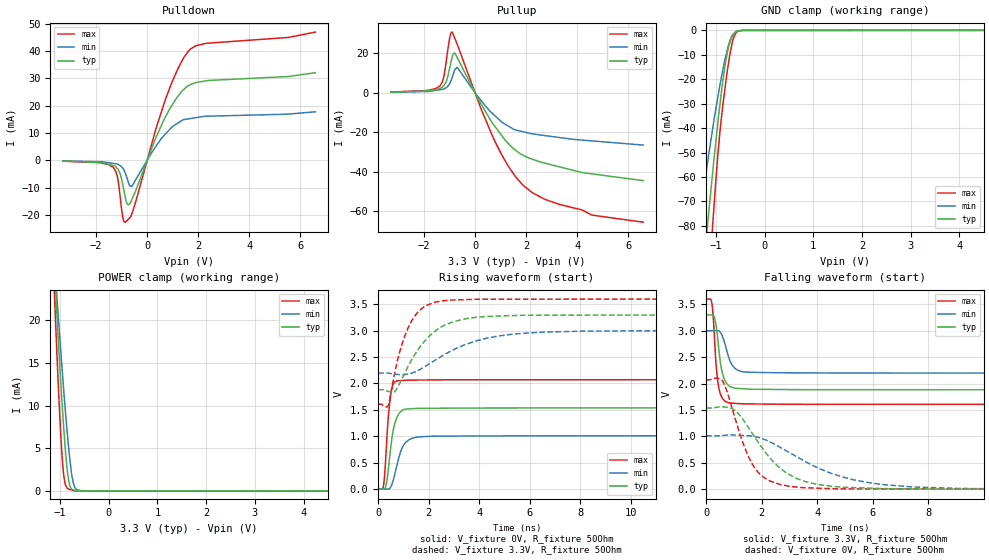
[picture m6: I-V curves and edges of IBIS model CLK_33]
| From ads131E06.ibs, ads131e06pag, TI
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|   CLK 3.3V Model
[Model]   CLK_33
Model_type   I/O
|for all products
|Signals   CLK
Vinl = 0.66
Vinh = 2.64
Vmeas = 1.65
Vref = 1.65
Cref = 2pF
Rref = 50
|   typ   min   max
|   (nom PVT)   (Fast PVT)   (slow PVT)
|C_comp from frequency sweep method (F=64MHz)
|   (HIGH Z)
|C_comp   3.0737920e-12   2.2794920e-12   3.8127910e-12
|   (ON state)
|C_comp   5.2867200e-12   4.2791250e-12   6.0292710e-12
|   (OFF state)
|C_comp   6.2204500e-12   5.1534470e-12   7.4413370e-12
|C_comp from LC tank measurement(L=1nH)
|   (HIGH Z)
|C_comp   2.430E-12   1.871E-12   3.021E-12
|   (ON state)
C_comp   2.536E-12   1.968E-12   3.105E-12
|   (OFF state)
|C_comp   2.524E-12   1.950E-12   3.148E-12
| Where   nom PVT is  Nominal Process, 3.3V, 27C
|   Fast PVT is Strong Process, 3.6V, -40C
|   Slow PVT is Weak Process, 3V, 85C
[Voltage Range]   3.3   3   3.6
[Temperature Range]   27   85   -40
[Pullup Reference]   3.3   3   3.6
[Pulldown Reference]   0   0   0
[Power Clamp Reference]   3.3   3   3.6
[GND Clamp Reference]   0   0   0
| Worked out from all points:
|   slope of the pulldown table from 0 to 0.495 V, typ, clamps not added: 43.2 ohm
|   slope of the pullup table from 0 to 0.495 V, typ, clamps not added: 43.3 ohm
|   GND clamp passes 1 mA (typ) near -0.61 V on its own axis
|   POWER clamp passes 1 mA (typ) near -0.81 V on its own axis
|   falling waveform, V_fixture 3.3V, R_fixture 50Ohm: 20-80 % time 223ps typ, 299ps min, 168ps max; typ from 3.3 V to 1.88 V
|   rising waveform, V_fixture 0V, R_fixture 50Ohm: 20-80 % time 266ps typ, 362ps min, 185ps max; typ from 0 V to 1.54 V
|   rising waveform, V_fixture 3.3V, R_fixture 50Ohm: 20-80 % time 1.3ns typ, 2.17ns min, 765ps max; typ from 1.88 V to 3.3 V
|   falling waveform, V_fixture 0V, R_fixture 50Ohm: 20-80 % time 1.45ns typ, 2.51ns min, 868ps max; typ from 1.54 V to 0 V
[Pulldown]
|   Voltage   I(typ)   I(min)   I(max)
-3.3V     -285.2uA   -205.1uA   -305.9uA
-1.334V   -1.903mA   -1.123mA   -2.529mA
-1.165V   -2.988mA   -1.357mA   -5.941mA
-1.06V    -4.818mA   -1.89mA    -13.08mA
-951.3mV  -9.091mA   -2.885mA   -21mA
-850.6mV  -13.69mA   -4.785mA   -22.61mA
-726.8mV  -16.25mA   -8.297mA   -21.49mA
-605.4mV  -14.49mA   -9.538mA   -19.68mA
711.2mV   15.74mA    9.54mA     22.12mA
1.215V    23.48mA    13.67mA    33.65mA
1.658V    27.46mA    15.21mA    40.4mA
6.59V     32.02mA    17.73mA    46.86mA
[GND Clamp]
|   Voltage   I(typ)   I(min)   I(max)
-3.3V     -585.9mA   -419.8mA   -805.2mA
-1.364V   -121.4mA   -81.78mA   -172mA
-1.248V   -96.06mA   -64.96mA   -135.3mA
-1.155V   -76.25mA   -51.89mA   -106.4mA
-1.067V   -58.43mA   -40.42mA   -80.04mA
-958.2mV  -37.75mA   -27.18mA   -50.79mA
-850.6mV  -19.87mA   -15.56mA   -29.67mA
-760.6mV  -8.736mA   -7.664mA   -16.07mA
-712.4mV  -5.071mA   -4.347mA   -9.829mA
-646mV    -1.87mA    -1.599mA   -3.719mA
-585.8mV  -599.8uA   -419.2uA   -1.094mA
6.59V     0A         0A         0A
[Pullup]
|   Voltage   I(typ)   I(min)   I(max)
-3.3V     365.8uA    284.3uA    421.3uA
-1.382V   2.277mA    1.572mA    3.466mA
-1.226V   3.655mA    1.921mA    8.042mA
-1.123V   5.876mA    2.679mA    16.58mA
-988.7mV  12.8mA     4.836mA    28.09mA
-909.9mV  17.35mA    7.374mA    30.76mA
-804.6mV  20.18mA    11.39mA    28mA
-682.5mV  17.49mA    12.65mA    24.05mA
725.1mV   -16.03mA   -10.92mA   -23.07mA
1.864V    -31.4mA    -19.61mA   -46.52mA
4.577V    -40.98mA   -24.29mA   -61.83mA
6.59V     -44.4mA    -26.41mA   -65.43mA
[POWER Clamp]
|   Voltage   I(typ)   I(min)   I(max)
-3.3V     287.9mA    235.1mA    365.7mA
-1.115V   26.05mA    26.93mA    23.11mA
-1.106V   25.05mA    26.15mA    21.77mA
-1.06V    20.17mA    22.41mA    15.6mA
-1.008V   14.97mA    18.22mA    9.117mA
-958.2mV  10.33mA    14.39mA    4.094mA
-909.9mV  6.299mA    10.79mA    1.292mA
-837.9mV  1.817mA    5.958mA    244uA
-769.9mV  272.5uA    2.326mA    127.7uA
-719.9mV  125.8uA    801.6uA    42.51uA
-544.6mV  5.214uA    4.036uA    6.182uA
6.59V     0A         0A         0A
[Ramp]
R_load = 50
|   typ   min   max
dV/dt_r   0.922226/2.64298e-010  0.605476/3.60315e-010   1.24254/1.85024e-010
dV/dt_f   0.851354/2.21748e-010  0.481827/2.9797e-010   1.19615/1.67153e-010
[Falling Waveform]
V_fixture = 3.3V
V_fixture_min = 3V
V_fixture_max = 3.6V
R_fixture = 50Ohm
C_fixture = 0F
|   Time   V(typ)   V(min)   V(max)
0s        3.3V       3V         3.6V
211.2ps   3.301V     3.002V     3.509V
260.7ps   3.291V     3.002V     3.219V
368.4ps   3.06V      3.003V     2.296V
468.3ps   2.599V     2.994V     1.894V
616.2ps   2.139V     2.857V     1.7V
813.5ps   1.959V     2.498V     1.635V
1.021ns   1.916V     2.295V     1.626V
1.446ns   1.898V     2.215V     1.615V
15.91ns   1.881V     2.197V     1.606V
[Rising Waveform]
V_fixture = 0V
V_fixture_min = 0V
V_fixture_max = 0V
R_fixture = 50Ohm
C_fixture = 0F
|   Time   V(typ)   V(min)   V(max)
0s        5.091uV    2.956uV    -113.5nV
210ps     -2.975mV   -2.493mV   60.96mV
329.7ps   116.6mV    -3.914mV   845.1mV
392.6ps   338.1mV    -4.661mV   1.322V
475ps     691.8mV    17.93mV    1.711V
577.4ps   1.069V     136.2mV    1.97V
736ps     1.348V     436.5mV    2.049V
1.083ns   1.514V     879.4mV    2.06V
1.609ns   1.527V     986.7mV    2.065V
15.91ns   1.537V     1.009V     2.071V
[Rising Waveform]
V_fixture = 3.3V
V_fixture_min = 3V
V_fixture_max = 3.6V
R_fixture = 50Ohm
C_fixture = 0F
|   Time   V(typ)   V(min)   V(max)
0s        1.881V     2.197V     1.606V
405.3ps   1.848V     2.195V     1.589V
638.2ps   1.838V     2.176V     2.159V
836.1ps   1.984V     2.168V     2.573V
1.304ns   2.43V      2.191V     3.17V
1.707ns   2.727V     2.279V     3.413V
2.244ns   2.989V     2.437V     3.538V
3.405ns   3.221V     2.729V     3.589V
5.443ns   3.288V     2.94V      3.597V
15.91ns   3.3V       3V         3.6V
[Falling Waveform]
|Gnd
V_fixture = 0V
V_fixture_min = 0V
V_fixture_max = 0V
R_fixture = 50Ohm
C_fixture = 0F
|   Time   V(typ)   V(min)   V(max)
0s        1.537V     1.009V     2.071V
590.5ps   1.56V      1.016V     2.049V
1.031ns   1.497V     1.025V     1.366V
1.322ns   1.325V     1.017V     883.3mV
1.639ns   1.074V     1.005V     497mV
2.056ns   752.9mV    949.3mV    230.9mV
2.661ns   398.9mV    793.4mV    89mV
3.981ns   92.96mV    414.1mV    19.4mV
6.308ns   11.96mV    90.43mV    4.708mV
15.91ns   5.091uV    2.956uV    -113.5nV
